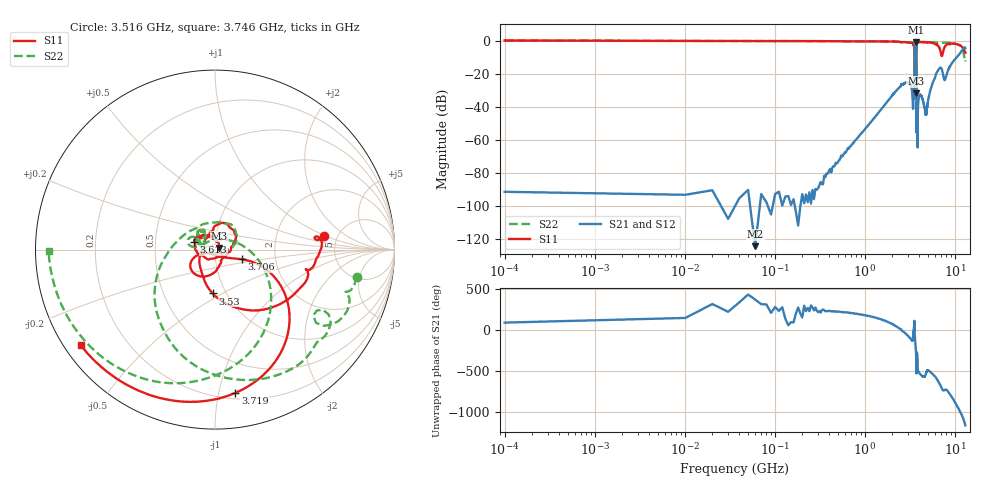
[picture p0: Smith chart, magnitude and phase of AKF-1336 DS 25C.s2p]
!Akoustis s2p Touchstone File
!Script Version: 1.0
!Creation Data: 5/11/2020 at 10:11 AM
!DEEMBEDDING STATE: ON
!DEMBEDDING OFFSET: 0.2 dB static
! Freq Mag(S11) Angle(S11)Mag(S21) Angle(S21)Mag(S12) Angle(S12)Mag(S22) Angle(S22)
# GHz S MA R 50
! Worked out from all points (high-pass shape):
!   11000 points, 100 kHz to 13 GHz, reference 50 ohm
!   highest |S21| = -0.87 dB at 3.662 GHz (marker M1); lowest = -124.2 dB at 60.4 MHz (marker M2)
!   |S21| within 3 dB of the highest: 3.538 GHz to 3.708 GHz (170.1 MHz wide, 4.7 % of centre); 12.72 GHz to 12.83 GHz (113.9 MHz wide, 0.892 % of centre)
!   lowest |S11| = -31.6 dB at 3.646 GHz (marker M3), VSWR 1.05, Z = 52.5 + j0.978 ohm
!   |S11| at or under -10 dB: 3.528 GHz to 3.709 GHz (180.7 MHz wide, 4.99 % of centre)
!   |S22| runs from -33.8 to 0.2 dB; largest |S21 - S12| = 0.0032
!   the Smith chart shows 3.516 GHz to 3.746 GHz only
!   S11 on the Smith chart (normalised r, x): 3.516 GHz: 3.90, +0.96; 3.53 GHz: 0.87, -0.45; 3.613 GHz: 0.79, +0.07; 3.706 GHz: 1.35, -0.15; 3.719 GHz: 0.25, -1.12; 3.746 GHz: 0.05, -0.32
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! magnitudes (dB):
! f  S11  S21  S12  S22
! 100 kHz  0.3  -91.3  -76.5  0.2
! 10.15 MHz  0.0  -93.1  -94.4  0.0
! 40.3 MHz  0.0  -95.1  -94.9  0.0
! 60.4 MHz  -0.1  -124.2  -95.9  0.0
! 261.4 MHz  -0.1  -90.2  -93.5  -0.1
! 1.829 GHz  -0.3  -35.7  -35.7  -0.3
! 3.036 GHz  -0.9  -25.0  -24.9  -0.8
! 3.415 GHz  -1.5  -40.5  -40.5  -1.1
! 3.516 GHz  -4.3  -22.5  -22.5  -1.9
! 3.53 GHz  -12.2  -12.6  -12.6  -4.1
! 3.579 GHz  -24.6  -1.3  -1.3  -28.6
! 3.613 GHz  -18.1  -1.3  -1.3  -18.0
! 3.646 GHz  -31.6  -1.1  -1.1  -20.9
! 3.662 GHz  -18.1  -0.9  -0.9  -19.4
! 3.706 GHz  -15.9  -3.1  -3.1  -23.8
! 3.719 GHz  -1.9  -21.1  -21.0  -2.2
! 3.746 GHz  -0.7  -43.1  -43.1  -0.7
! 3.829 GHz  -0.6  -63.6  -63.3  -0.5
! 4.018 GHz  -0.7  -32.9  -32.9  -0.6
! 4.753 GHz  -0.9  -44.7  -44.7  -0.7
! 6.423 GHz  -2.7  -18.1  -18.1  -1.2
! 13 GHz  -7.1  -4.4  -4.4  -11.8
